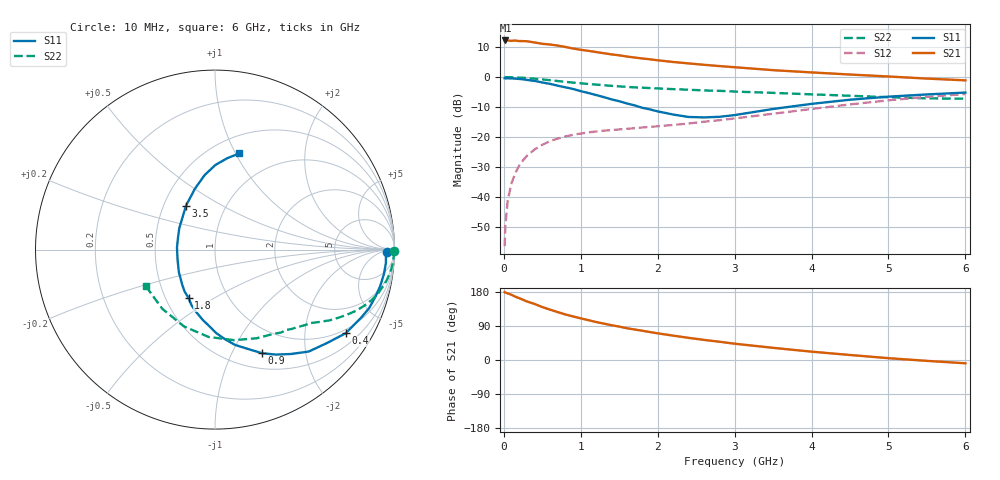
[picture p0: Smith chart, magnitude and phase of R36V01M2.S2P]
! SIEMENS Small Signal Semiconductors
! BFR181
! Si NPN RF Bipolar Junction Transistor in SOT23
! VCE = 6 V  IC = 1.2 mA
! Common Emitter S-Parameters:  May  1996
# GHz  S  MA  R  50
!  f  S11  S21  S12  S22
! GHz  MAG  ANG  MAG  ANG  MAG  ANG  MAG  ANG
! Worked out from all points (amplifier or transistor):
!   36 points, 10 MHz to 6 GHz, reference 50 ohm
!   highest |S21| = 12.2 dB at 20 MHz (marker M1)
!   |S21| within 3 dB of that: start of sweep to 971.6 MHz
!   unconditionally stable (mu >= 1): 1.955 GHz to 3.637 GHz
!   at 250 MHz: K = 0.17, MSG = 19.9 dB, |S12| = -27.8 dB
!   at 1.4 GHz: K = 0.81, MSG = 12.7 dB, |S12| = -17.7 dB
!   at 6 GHz: K = 0.86, MSG = 2.3 dB, |S12| = -5.6 dB
!   S11 on the Smith chart (normalised r, x): 10 MHz: 41, -13; 400 MHz: 0.87, -3.20; 900 MHz: 0.68, -1.31; 1.8 GHz: 0.65, -0.39; 3.5 GHz: 0.65, +0.35; 6 GHz: 0.67, +1.03
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0.01  0.9567 -0.8  4.049 179.3  0.0015 92.1  0.9977 -0.4
0.02  0.9528 -1.6  4.095 178.1  0.0033 91.2  0.9979 -0.9
0.05  0.9552 -4.4  4.078 175.8  0.0087 88.1  0.9966 -2.0
0.1  0.9511 -8.2  4.038 172.0  0.0169 83.5  0.9944 -3.9
0.15  0.9424 -12.5  4.075 166.9  0.0252 81.7  0.9884 -6.1
0.3  0.8981 -25.0  3.972 154.5  0.0485 74.4  0.9633 -11.6
0.4  0.8647 -32.6  3.788 147.8  0.0618 69.7  0.9415 -15.0
0.5  0.8134 -39.7  3.599 139.7  0.074 65.7  0.9162 -17.9
0.6  0.7716 -47.4  3.505 132.9  0.0851 61.7  0.8885 -20.6
0.7  0.719 -54.0  3.365 126.5  0.094 58.6  0.8605 -23.1
0.9  0.6337 -65.6  3 114.9  0.1087 53.7  0.8099 -27.0
1.1  0.5427 -78.1  2.744 105.1  0.1194 50.2  0.7678 -30.3
1.4  0.4246 -94.8  2.394 91.8  0.13 47.4  0.7149 -34.3
1.6  0.3628 -106.9  2.207 83.8  0.1369 47.0  0.6871 -36.3
1.8  0.3071 -118.7  2.047 77.2  0.1443 47.0  0.6653 -38.5
2.2  0.2372 -148.1  1.79 64.3  0.1588 48.8  0.6297 -43.3
2.6  0.2122 176.7  1.607 53.1  0.1797 50.8  0.5992 -48.4
3  0.2321 149.0  1.463 43.0  0.2042 52.2  0.5737 -54.7
3.5  0.2937 123.3  1.306 32.1  0.2443 52.2  0.5454 -65.0
4.5  0.4193 97.9  1.104 13.2  0.3497 46.9  0.4879 -94.2
5.5  0.5136 82.4  0.945 -2.3  0.4677 34.7  0.4416 -131.7
6  0.5521 75.9  0.883 -8.7  0.5221 27.1  0.4359 -152.0
